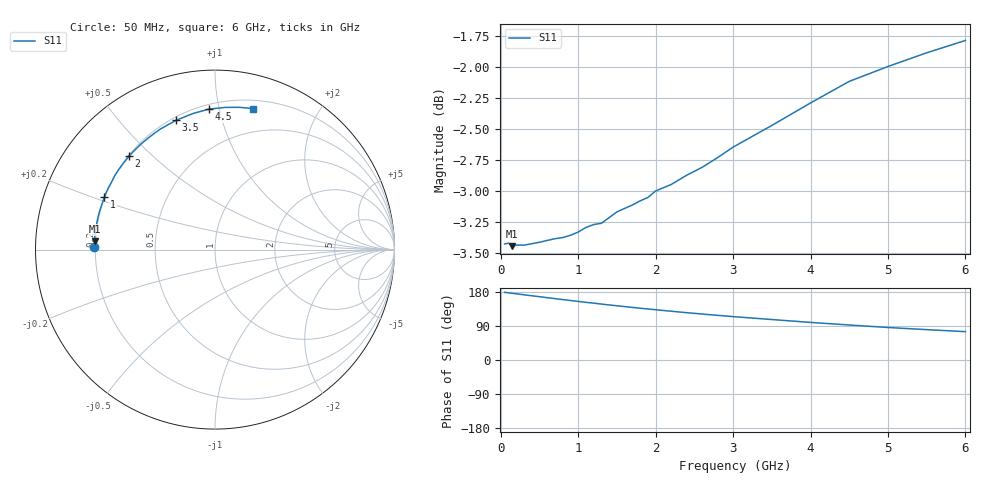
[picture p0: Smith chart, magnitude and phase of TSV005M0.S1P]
! SIEMENS Small Signal Semiconductors
! BAT14-03W
! Si Schottky Diode in SOD323
! IF = 5 mA
! S-Parameters:  November  1995
# GHz  S  MA  R  50
!  f  S11
! GHz  MAG  ANG
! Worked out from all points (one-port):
!   34 points, 50 MHz to 6 GHz, reference 50 ohm
!   lowest |S11| = -3.4 dB at 150 MHz (marker M1), VSWR 5.11, Z = 9.79 + j1.68 ohm
!   |S11| at or under -10 dB: nowhere
!   S11 on the Smith chart (normalised r, x): 50 MHz: 0.19, +0.01; 1 GHz: 0.20, +0.22; 2 GHz: 0.20, +0.42; 3.5 GHz: 0.22, +0.72; 4.5 GHz: 0.23, +0.93; 6 GHz: 0.27, +1.27
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0.05  0.6741 178.7
0.1  0.6747 177.3
0.15  0.6728 176.0
0.2  0.6734 174.8
0.4  0.6743 169.5
0.5  0.6752 167.1
0.7  0.6774 162.0
0.8  0.6782 159.5
0.9  0.6796 157.0
1  0.6816 154.7
1.1  0.6845 152.2
1.2  0.6864 150.0
1.3  0.6872 147.6
1.4  0.6908 145.3
1.5  0.6945 143.1
1.6  0.6967 140.9
1.8  0.7016 136.6
2  0.708 132.7
2.2  0.7123 128.7
2.4  0.7184 124.9
2.8  0.7302 117.8
3  0.7373 114.5
3.5  0.7523 106.8
4  0.7681 99.2
4.5  0.7836 92.4
5  0.7945 85.8
5.5  0.8046 80.1
6  0.8139 74.8
